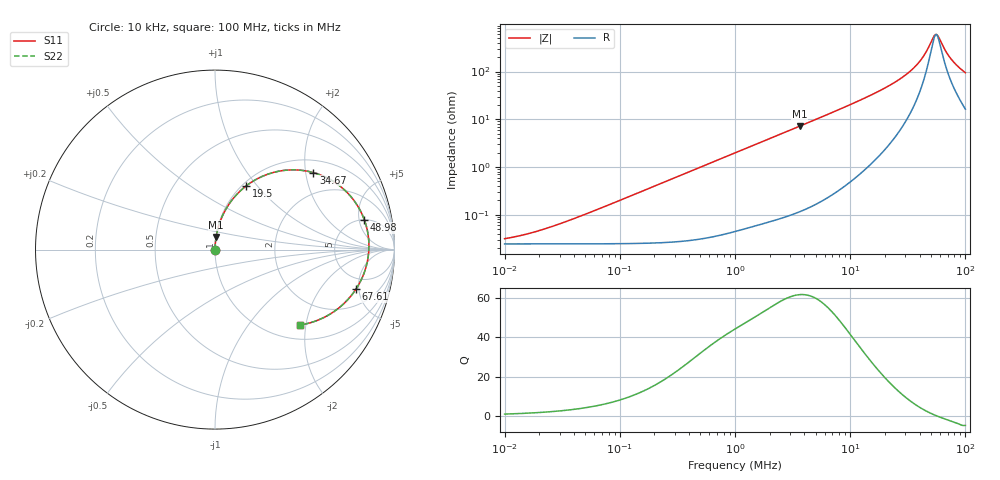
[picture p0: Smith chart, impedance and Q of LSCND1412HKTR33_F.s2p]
! LSCND1412HKTR33_F  S-PARAMETER MODEL  ( Standard Model )
! Model Generated by TAIYO YUDEN Corporation (http://www.ty-top.com)
! Version 2.0
! TAIYO YUDEN Control No. 220720
! Copyright(c) 2022 TAIYO YUDEN CO.,LTD. All Rights Reserved.
! Product Description (link to TY-COMPAS)
! https://ds.yuden.co.jp/TYCOMPAS/or/detail?pn=LSCND1412HKTR33MF&u=M
! Products Name : Inductors
! Characteristics :
!  Inductance : 0.33 [uH] , SRF(min) : - [Hz] , DC Resistance(max) : 27 [mOhm]
!  Rated Current : Saturation  5.4 [A] (dL = 30 [%]), Temp Rise  4.0 [A] (dT = 40 [degC])
!  Case Size : 1.4 x 1.2 / 0.055 x 0.047 [mm/inch] , Thickness : 0.8 / 0.031 [mm/inch]
!  (Conditions: Temperature = 25 [degC] , DC Bias Current = 0 [A])
! External Node Assignments :
!  1  o---GGG---o  2
! GND o---------o GND
! Frequency Range : 10kHz  -  100MHz  [ 402 STEP ]
# MHz S RI R 50
! Freq[MHz].  S11 Real  S11 Imag  S21 Real  S21 Imag  S12 Real  S12 Imag  S22 Real  S22 Imag
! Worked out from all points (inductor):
!   401 points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, 10 kHz to 100 MHz, reference 50 ohm
!   read as one part in series: L = 317 nH near 37.15 kHz
!   highest Q = 61.9 at 3.631 MHz (marker M1), where L = 314 nH
!   self-resonance near 55.81 MHz
!   S11 on the Smith chart (normalised r, x): 10 kHz: 1.00, +0.00; 19.5 MHz: 1.04, +0.87; 34.67 MHz: 1.33, +2.21; 48.98 MHz: 5.04, +5.96; 67.61 MHz: 3.54, -4.66; 100 MHz: 1.33, -1.86
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0.01  0.000246 0.000199  0.9998 -0.000199  0.9998 -0.000199  0.000246 0.000199
0.019953  0.000246 0.000397  0.9998 -0.000397  0.9998 -0.000397  0.000246 0.000397
0.046774  0.000247 0.000931  0.9998 -0.000931  0.9998 -0.000931  0.000247 0.000931
0.218776  0.000278 0.00435  0.9997 -0.00435  0.9997 -0.00435  0.000278 0.00435
1  0.000838 0.0198  0.9992 -0.0198  0.9992 -0.0198  0.000838 0.0198
3.630781  0.00623 0.071  0.9938 -0.071  0.9938 -0.071  0.00623 0.071
4.677351  0.00994 0.0913  0.9901 -0.0913  0.9901 -0.0913  0.00994 0.0913
11.22019  0.0552 0.2154  0.9448 -0.2154  0.9448 -0.2154  0.0552 0.2154
19.49845  0.1725 0.3539  0.8275 -0.3539  0.8275 -0.3539  0.1725 0.3539
21.87762  0.2196 0.3857  0.7804 -0.3857  0.7804 -0.3857  0.2196 0.3857
28.84032  0.3879 0.4416  0.6121 -0.4416  0.6121 -0.4416  0.3879 0.4416
34.67368  0.5485 0.4288  0.4515 -0.4288  0.4515 -0.4288  0.5485 0.4288
41.68694  0.7223 0.3317  0.2777 -0.3317  0.2777 -0.3317  0.7223 0.3317
45.70882  0.7939 0.2447  0.2061 -0.2447  0.2061 -0.2447  0.7939 0.2447
48.97788  0.8323 0.1656  0.1677 -0.1656  0.1677 -0.1656  0.8323 0.1656
53.70318  0.8567 0.0494  0.1433 -0.0494  0.1433 -0.0494  0.8567 0.0494
56.23413  0.8567 -0.00976  0.1433 0.00976  0.1433 0.00976  0.8567 -0.00976
58.88437  0.8488 -0.0675  0.1512 0.0675  0.1512 0.0675  0.8488 -0.0675
67.6083  0.7854 -0.2204  0.2146 0.2204  0.2146 0.2204  0.7854 -0.2204
74.13102  0.7205 -0.2985  0.2795 0.2985  0.2795 0.2985  0.7205 -0.2985
81.28305  0.6466 -0.3561  0.3534 0.3561  0.3534 0.3561  0.6466 -0.3561
100  0.4759 -0.4196  0.5241 0.4196  0.5241 0.4196  0.4759 -0.4196
